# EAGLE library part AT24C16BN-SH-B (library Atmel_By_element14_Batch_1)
Two-wire Serial EEPROM
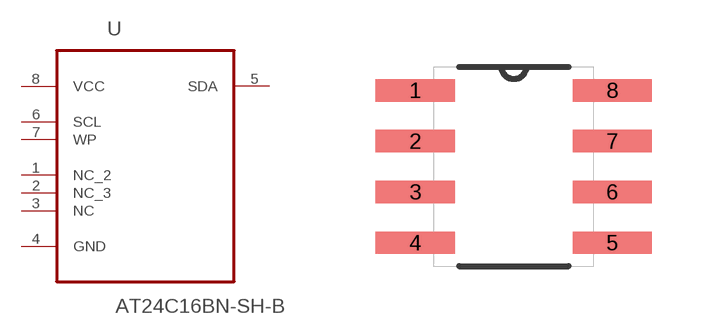
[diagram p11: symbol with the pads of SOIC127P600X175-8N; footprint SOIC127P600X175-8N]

Designator prefix U

## AT24C16BN-SH-B (MPN: AT24C16BN-SH-B; OC_FARNELL: 1362651; OC_NEWARK: 50M3324; PACKAGE: SOIC-8; SUPPLIER: Atmel)  [SOIC127P600X175-8N]
1  NC_2  nc
2  NC_3  nc
3  NC  nc
4  GND  pas
5  SDA
6  SCL  in
7  WP  in
8  VCC  pwr

## Footprint SOIC127P600X175-8N (pad centres in mm)
smd 1.981 x 0.559: 1 -2.464,1.905; 2 -2.464,0.635; 3 -2.464,-0.635; 4 -2.464,-1.905; 5 2.464,-1.905; 6 2.464,-0.635; 7 2.464,0.635; 8 2.464,1.905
